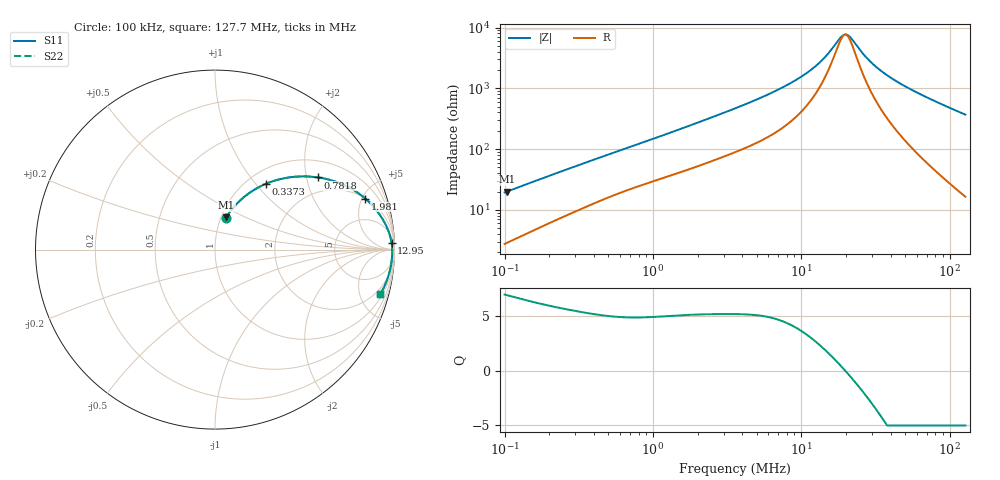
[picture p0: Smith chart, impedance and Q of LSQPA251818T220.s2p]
! LSQPA251818T220  S-PARAMETER MODEL  ( General Type )
! Model Generated by TAIYO YUDEN Corporation (http://www.ty-top.com)
! Version 2.0
! TAIYO YUDEN Control No. 100810NF25SB-FAC
! Copyright(c) 2007 TAIYO YUDEN CO.,LTD. All Rights Reserved.
! Product Description (link to TY-COMPAS)
! https://ds.yuden.co.jp/TYCOMPAS/or/detail?pn=LSQPA251818T220K&u=M
! Products Name : Inductors
! Characteristics :
!  Inductance : 22 uH , SRF(min) : 19 MHz , DC Resistance(max) : 1.001 Ohm
!  Rated Current : Saturation :320 mA , Temp Rise : 460 mA (40 degC)
!  Case Size : 2.5 x 1.8 / 0.098 x 0.071 [mm/inch] , Thickness : 1.8 / 0.071 [mm/inch]
!  (Conditions: Temperature = 25 degC , DC Bias Current/Voltage = 0A / 0V)
! External Node Assignments :
!  1  o---GGG---o  2
! GND o---------o GND
! Frequency Range : 0.1MHz  -  127.746476MHz  [ 402 STEP ]
# MHz S RI R 50
! Freq[MHz].  S11 Real  S11 Imag  S21 Real  S21 Imag  S12 Real  S12 Imag  S22 Real  S22 Imag
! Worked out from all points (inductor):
!   401 points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, 100 kHz to 127.7 MHz, reference 50 ohm
!   read as one part in series: L = 29.8 uH near 103.6 kHz
!   highest Q = 6.89 at 103.6 kHz (marker M1), where L = 30.4 uH
!   self-resonance near 19.78 MHz
!   S11 on the Smith chart (normalised r, x): 100 kHz: 1.06, +0.38; 337.3 kHz: 1.21, +1.14; 781.8 kHz: 1.48, +2.33; 1.981 MHz: 2.03, +5.30; 12.95 MHz: 20, +46; 127.7 MHz: 1.33, -7.37
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0.1  0.0594 0.1752  0.9406 -0.1752  0.9406 -0.1752  0.0594 0.1752
0.103641  0.0626 0.1803  0.9374 -0.1803  0.9374 -0.1803  0.0626 0.1803
0.190358  0.1443 0.2777  0.8557 -0.2777  0.8557 -0.2777  0.1443 0.2777
0.33137  0.2796 0.3649  0.7204 -0.3649  0.7204 -0.3649  0.2796 0.3649
0.337349  0.2849 0.3671  0.7151 -0.3671  0.7151 -0.3671  0.2849 0.3671
0.518156  0.427 0.4041  0.573 -0.4041  0.573 -0.4041  0.427 0.4041
0.781763  0.5723 0.4023  0.4277 -0.4023  0.4277 -0.4023  0.5723 0.4023
1.098062  0.6852 0.374  0.3148 -0.374  0.3148 -0.374  0.6852 0.374
1.981074  0.8372 0.2843  0.1628 -0.2843  0.1628 -0.2843  0.8372 0.2843
3.574164  0.9232 0.1866  0.0768 -0.1866  0.0768 -0.1866  0.9232 0.1866
7.308182  0.9703 0.0924  0.0297 -0.0924  0.0297 -0.0924  0.9703 0.0924
9.556469  0.9785 0.0642  0.0215 -0.0642  0.0215 -0.0642  0.9785 0.0642
11.84371  0.9827 0.0439  0.0173 -0.0439  0.0173 -0.0439  0.9827 0.0439
12.95142  0.984 0.0359  0.016 -0.0359  0.016 -0.0359  0.984 0.0359
14.94322  0.9855 0.0235  0.0145 -0.0235  0.0145 -0.0235  0.9855 0.0235
18.51973  0.9869 0.00547  0.0131 -0.00547  0.0131 -0.00547  0.9869 0.00547
20.25182  0.9872 -0.00198  0.0128 0.00198  0.0128 0.00198  0.9872 -0.00198
21.75342  0.9873 -0.00797  0.0127 0.00797  0.0127 0.00797  0.9873 -0.00797
28.95886  0.9868 -0.0327  0.0132 0.0327  0.0132 0.0327  0.9868 -0.0327
39.24654  0.9843 -0.0618  0.0157 0.0618  0.0157 0.0618  0.9843 -0.0618
64.7509  0.9729 -0.1227  0.0271 0.1227  0.0271 0.1227  0.9729 -0.1227
127.7465  0.922 -0.2468  0.078 0.2468  0.078 0.2468  0.922 -0.2468
